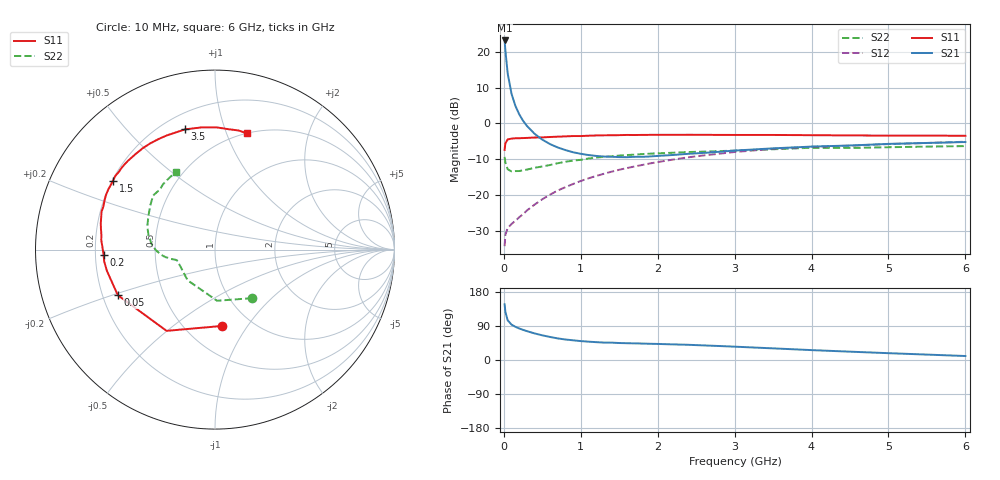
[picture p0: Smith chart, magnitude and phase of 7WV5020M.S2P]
! Infineon Technologies  Discrete & RF Semiconductors
! BFS17W
! Si NPN RF Bipolar Junction Transistor in SOT323
! VCE = 0.5 V  IC = 20 mA
! Common Emitter S-Parameters:  August  1999
# GHz  S  MA  R  50
!  f  S11  S21  S12  S22
! GHz  MAG  ANG  MAG  ANG  MAG  ANG  MAG  ANG
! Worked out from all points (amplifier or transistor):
!   36 points, 10 MHz to 6 GHz, reference 50 ohm
!   highest |S21| = 23.1 dB at 10 MHz (marker M1)
!   |S21| within 3 dB of that: start of sweep to 21.13 MHz
!   unconditionally stable (mu >= 1): start of sweep to end of sweep
!   at 250 MHz: K = 4.99, MAG = 3.1 dB, |S12| = -25.3 dB
!   at 1.4 GHz: K = 3.44, MAG = -6.2 dB, |S12| = -13.5 dB
!   at 6 GHz: K = 1.16, MAG = -2.5 dB, |S12| = -5.1 dB
!   S11 on the Smith chart (normalised r, x): 10 MHz: 0.74, -0.77; 50 MHz: 0.26, -0.21; 200 MHz: 0.23, -0.02; 1.5 GHz: 0.20, +0.30; 3.5 GHz: 0.29, +0.74; 6 GHz: 0.50, +1.18
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0.01  0.4272 -84.4  14.36 147.0  0.0194 56.6  0.341 -52.5
0.02  0.527 -120.8  10.45 126.8  0.028 40.6  0.2852 -87.7
0.05  0.5981 -154.9  4.979 104.7  0.0346 28.7  0.2292 -131.8
0.1  0.6136 -168.8  2.587 93.4  0.0396 30.9  0.2143 -153.2
0.15  0.6208 -173.9  1.757 87.6  0.0438 37.3  0.2164 -159.7
0.2  0.6211 -177.1  1.34 83.2  0.0491 43.2  0.2167 -162.5
0.25  0.6248 -179.9  1.089 79.5  0.0542 46.9  0.2217 -164.7
0.3  0.6277 178.6  0.923 76.2  0.061 50.2  0.2269 -165.5
0.4  0.6358 175.2  0.716 70.1  0.0738 54.6  0.2405 -167.1
0.5  0.639 172.3  0.594 65.1  0.0875 57.8  0.2509 -167.9
0.6  0.6461 169.6  0.515 60.8  0.1014 59.5  0.2628 -169.7
0.7  0.6533 166.9  0.462 57.0  0.1158 60.4  0.2782 -171.3
0.9  0.6663 161.6  0.396 52.0  0.1428 61.2  0.3027 -174.8
1.1  0.6736 156.0  0.362 48.4  0.1714 60.4  0.3238 -178.4
1.5  0.6861 145.9  0.339 44.8  0.2257 57.5  0.3557 174.7
2.2  0.6923 129.7  0.363 41.2  0.3132 50.2  0.3902 163.7
2.8  0.6916 117.0  0.402 36.9  0.378 43.1  0.411 155.0
3.5  0.6903 104.0  0.449 30.7  0.442 34.5  0.4357 146.0
4  0.685 96.4  0.475 26.1  0.4718 28.4  0.4577 138.9
4.5  0.6808 89.2  0.492 22.0  0.4888 23.5  0.4548 132.1
5.5  0.6765 78.7  0.534 14.3  0.5331 15.4  0.4747 122.1
6  0.6715 74.6  0.55 10.5  0.5551 11.4  0.4826 116.6
